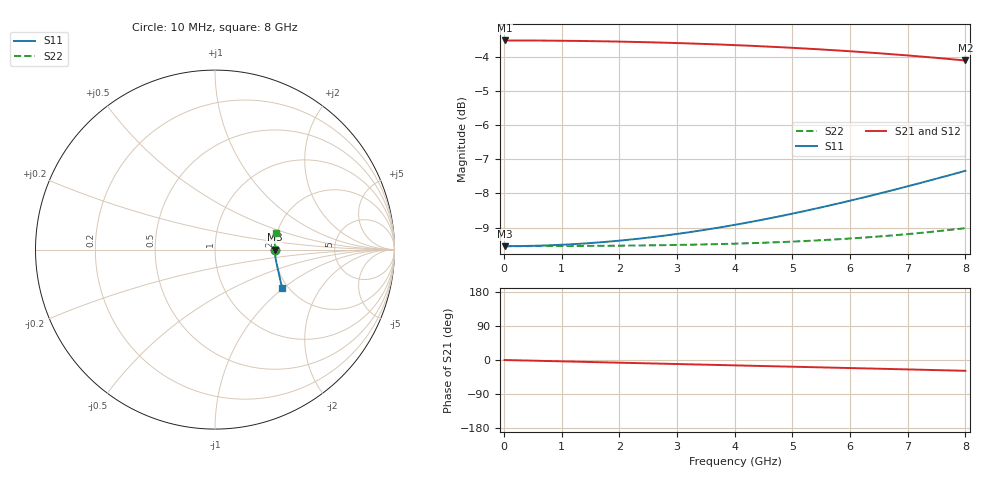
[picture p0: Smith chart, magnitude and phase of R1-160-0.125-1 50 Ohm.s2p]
!version-2
!date-03.2021
# MHz S RI R 50
!Freq ReS11 ImS11 ReS21 ImS21 ReS12 ImS12 ReS22 ImS22
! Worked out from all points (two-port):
!   800 points, 10 MHz to 8 GHz, reference 50 ohm
!   highest |S21| = -3.52 dB at 10 MHz (marker M1); lowest = -4.1 dB at 8 GHz (marker M2)
!   |S21| within 3 dB of the highest: start of sweep to end of sweep
!   lowest |S11| = -9.5 dB at 10 MHz (marker M3), VSWR 2.00, Z = 100 - j0.0481 ohm
!   |S11| at or under -10 dB: nowhere
!   |S22| runs from -9.5 to -9.0 dB; largest |S21 - S12| = 0
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10  0.3333 -0.000214  0.6667 -0.000407  0.6667 -0.000407  0.3333 9.64e-05
50  0.3333 -0.00107  0.6667 -0.00203  0.6667 -0.00203  0.3333 0.000482
680  0.3337 -0.0146  0.6658 -0.0276  0.6658 -0.0276  0.3333 0.00657
1010  0.3342 -0.0217  0.6648 -0.041  0.6648 -0.041  0.3333 0.00978
1350  0.3349 -0.0291  0.6633 -0.0548  0.6633 -0.0548  0.3333 0.0131
1680  0.3358 -0.0363  0.6614 -0.0681  0.6614 -0.0681  0.3333 0.0164
2010  0.3368 -0.0437  0.6591 -0.0813  0.6591 -0.0813  0.3333 0.0197
2340  0.338 -0.0512  0.6564 -0.0945  0.6564 -0.0945  0.3333 0.023
2680  0.3394 -0.059  0.6532 -0.108  0.6532 -0.108  0.3333 0.0266
3010  0.341 -0.0668  0.6497 -0.121  0.6497 -0.121  0.3334 0.03
3340  0.3426 -0.0747  0.6458 -0.1339  0.6458 -0.1339  0.3334 0.0336
3670  0.3444 -0.0828  0.6414 -0.1467  0.6414 -0.1467  0.3335 0.0372
4010  0.3464 -0.0914  0.6365 -0.1598  0.6365 -0.1598  0.3337 0.041
4670  0.3505 -0.1088  0.6258 -0.1847  0.6258 -0.1847  0.3341 0.0487
5000  0.3527 -0.1179  0.6198 -0.1968  0.6198 -0.1968  0.3344 0.0526
5340  0.3551 -0.1275  0.6133 -0.2092  0.6133 -0.2092  0.3347 0.0568
6000  0.3597 -0.147  0.5993 -0.2326  0.5993 -0.2326  0.3357 0.0653
6670  0.3643 -0.168  0.5836 -0.2554  0.5836 -0.2554  0.3372 0.0743
7050  0.3669 -0.1805  0.5739 -0.2679  0.5739 -0.2679  0.3382 0.0796
7440  0.3694 -0.1938  0.5635 -0.2802  0.5635 -0.2802  0.3395 0.0852
7960  0.3726 -0.2122  0.5488 -0.2961  0.5488 -0.2961  0.3415 0.0928
8000  0.3728 -0.2137  0.5477 -0.2973  0.5477 -0.2973  0.3417 0.0934
